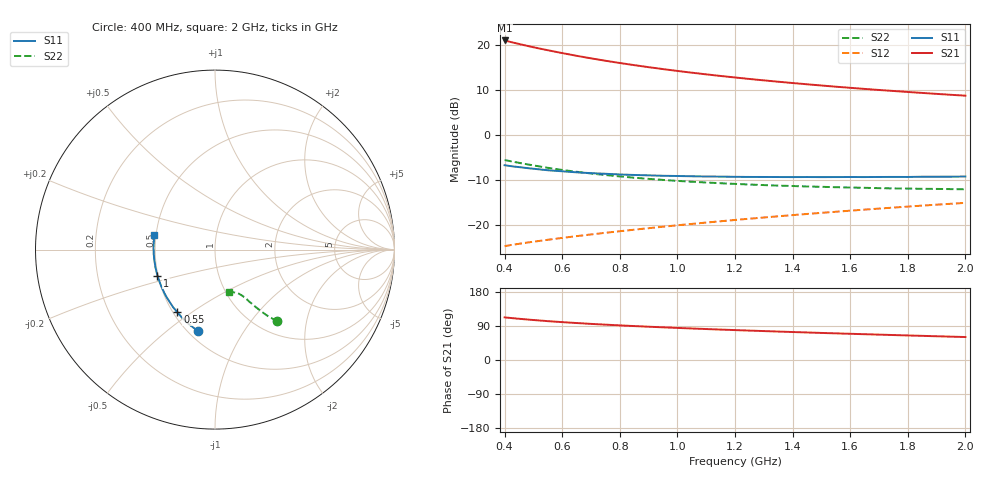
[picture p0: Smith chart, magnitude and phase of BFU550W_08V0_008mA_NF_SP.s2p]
! Filename:  P:\Prog\Test\Noise\ATS_data\Testdata_Net\06 Compressed Noise after Statistics\BFU550W_APM2013_11_D05_08p0V_008mA_NF_CM01_D.sf
! Date/Time: Tue 26/Mar/2013 16:25:24
! BFU550W_APM2013_11_D05_08p0V_1to35mA_NF_CM01_Bias5_R.sf
! Noise Parameter Data File
! BFU550W_APM2013_11_D05_08p0V_1to35mA_NF_CM01
! Date/time: Mon Mar 25 14:39:45 2013
! VAR V_out= 8.000000
! VAR I_out= 7.990000
! VAR V_in= 0.808700
! VAR I_in= 0.079600
! Device data file deembeded for feedlines and parallel
! Original file: \06 Compressed Noise after Statistics\BFU550W_APM2013_11_D05_08p0V_008mA_NF_CM01_R.sf
! Feed-files: PR019V01_070313_Feed1.s2p, PR019V01_070313_Feed2.s2p
! Parallel-file: PR019V01_070313_Par.s2p
# MHz S MA R 50
!  Freq-MHz  S11-mag  S11-arg  S21-mag  S21-arg  S12-mag  S12-arg  S22-mag  S22-arg
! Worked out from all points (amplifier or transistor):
!   37 points, 400 MHz to 2 GHz, reference 50 ohm
!   highest |S21| = 21.0 dB at 400 MHz (marker M1)
!   |S21| within 3 dB of that: start of sweep to 616.6 MHz
!   unconditionally stable (mu >= 1): 1.521 GHz to end of sweep
!   at 500 MHz: K = 0.67, MSG = 21.5 dB, |S12| = -23.6 dB
!   at 1.1 GHz: K = 0.94, MSG = 16.4 dB, |S12| = -19.4 dB
!   at 2 GHz: K = 1.02, MAG = 11.1 dB, |S12| = -15.0 dB
!   lowest NFmin = 0.65 dB at 420 MHz
!   S11 on the Smith chart (normalised r, x): 400 MHz: 0.56, -0.65; 550 MHz: 0.53, -0.44; 1 GHz: 0.50, -0.16; 2 GHz: 0.49, +0.09
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400  0.4629 -101.8  11.17 112.5  0.05873 56.5  0.529 -48.9
420  0.4533 -104.8  10.77 111.0  0.06028 56.3  0.5139 -49.6
440  0.4451 -107.5  10.39 109.5  0.06168 56.2  0.4993 -50.3
460  0.4378 -110.2  10.04 108.1  0.06309 56.1  0.4857 -50.9
500  0.4234 -115.3  9.392 105.5  0.06578 56.1  0.4608 -52.0
550  0.4074 -120.9  8.705 102.5  0.06911 56.3  0.4336 -53.1
600  0.3967 -126.1  8.091 99.9  0.0725 56.6  0.4104 -53.9
650  0.3862 -130.7  7.55 97.6  0.07584 56.9  0.392 -54.7
700  0.3784 -135.2  7.077 95.3  0.07921 57.3  0.375 -55.4
750  0.3723 -139.1  6.657 93.3  0.08257 57.7  0.3605 -55.9
800  0.3659 -143.0  6.284 91.4  0.086 58.0  0.3483 -56.6
850  0.3612 -146.6  5.951 89.5  0.08944 58.4  0.3366 -57.0
950  0.3538 -152.7  5.38 86.2  0.09646 59.2  0.3184 -58.0
1000  0.3518 -155.6  5.134 84.7  0.1 59.5  0.3104 -58.3
1100  0.3473 -160.9  4.704 81.7  0.1072 60.1  0.2979 -59.5
1200  0.3445 -165.7  4.344 78.9  0.1146 60.5  0.2877 -60.6
1250  0.3434 -168.1  4.182 77.6  0.1183 60.7  0.283 -61.0
1350  0.3426 -172.1  3.898 75.1  0.1259 61.0  0.2753 -62.2
1500  0.3418 -178.0  3.539 71.4  0.1374 61.3  0.267 -64.2
1650  0.3423 176.7  3.244 68.0  0.1492 61.3  0.2602 -66.2
1750  0.3436 173.7  3.079 65.9  0.1572 61.3  0.2562 -67.7
2000  0.3474 166.1  2.731 60.6  0.1773 60.8  0.2506 -72.1
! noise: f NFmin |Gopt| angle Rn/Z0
400  0.6716  0.06761  100.2  0.0802
460  0.6815  0.07587  105.1  0.0803
600  0.7101  0.0816  109.7  0.0848
800  0.7548  0.1278  125.6  0.0758
1000  0.753  0.159  137  0.0732
1200  0.8116  0.184  143.6  0.0712
1400  0.8402  0.2147  154.7  0.0665
1600  0.8126  0.2415  164.4  0.0654
1800  0.8666  0.269  173.8  0.0642
2000  0.9137  0.2989  -178  0.0595
